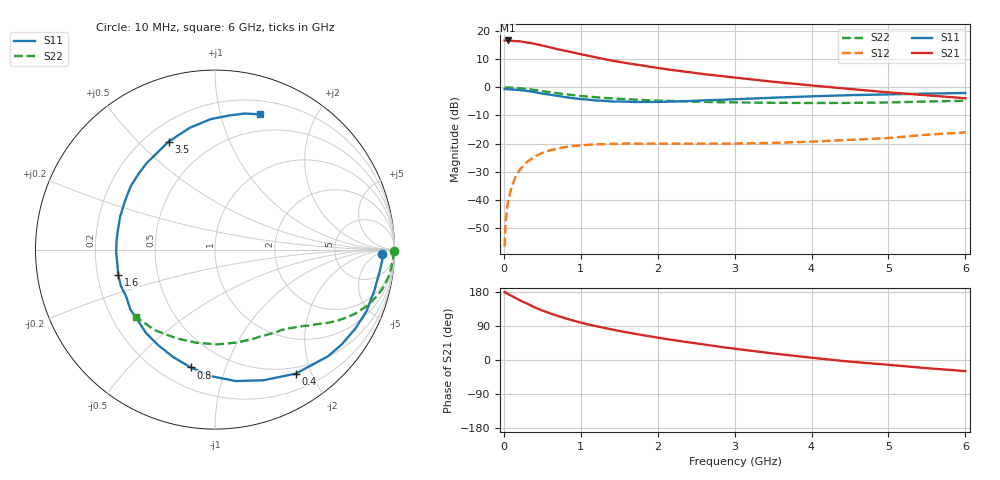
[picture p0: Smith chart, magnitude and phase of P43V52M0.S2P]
! SIEMENS Small Signal Semiconductors
! BFP182
! Si NPN RF Bipolar Junction Transistor in SOT143
! VCE = 3.5 V  IC = 2 mA
! Common Emitter S-Parameters:  March  1996
# GHz  S  MA  R  50
!  f  S11  S21  S12  S22
! GHz  MAG  ANG  MAG  ANG  MAG  ANG  MAG  ANG
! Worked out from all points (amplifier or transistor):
!   36 points, 10 MHz to 6 GHz, reference 50 ohm
!   highest |S21| = 16.7 dB at 50 MHz (marker M1)
!   |S21| within 3 dB of that: start of sweep to 680.8 MHz
!   unconditionally stable (mu >= 1): 2.2 GHz to 5.913 GHz
!   at 250 MHz: K = 0.12, MSG = 22.1 dB, |S12| = -27.9 dB
!   at 1.4 GHz: K = 0.68, MSG = 14.8 dB, |S12| = -20.1 dB
!   at 6 GHz: K = 0.99, MSG = 6.1 dB, |S12| = -16.0 dB
!   lowest NFmin = 1.10 dB at 450 MHz
!   S11 on the Smith chart (normalised r, x): 10 MHz: 25, -9; 400 MHz: 0.41, -1.77; 800 MHz: 0.32, -0.76; 1.6 GHz: 0.29, -0.12; 3.5 GHz: 0.29, +0.62; 6 GHz: 0.33, +1.33
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0.01  0.9308 -1.4  6.803 179.2  0.0015 85.8  0.9974 -0.5
0.02  0.9348 -3.1  6.801 178.4  0.0035 84.3  0.9896 -1.1
0.05  0.9259 -7.5  6.829 174.6  0.0088 88.7  0.9939 -2.8
0.1  0.9166 -14.7  6.738 169.3  0.0168 80.6  0.9872 -5.8
0.2  0.8968 -29.6  6.618 158.5  0.033 72.8  0.9678 -11.4
0.25  0.8817 -36.8  6.437 153.4  0.0401 68.8  0.953 -14.0
0.4  0.8248 -56.9  5.955 139.1  0.0588 58.0  0.8991 -20.7
0.5  0.7763 -69.7  5.545 130.5  0.0686 51.4  0.8582 -24.6
0.6  0.7414 -81.0  5.166 123.2  0.0759 46.0  0.8203 -27.7
0.7  0.7064 -91.5  4.759 116.4  0.0821 41.4  0.7876 -30.2
0.8  0.6705 -101.6  4.464 110.0  0.0869 36.8  0.7563 -32.5
0.9  0.6421 -111.4  4.178 104.1  0.0908 33.6  0.7288 -34.4
1.1  0.603 -129.6  3.654 93.6  0.0953 27.8  0.6834 -37.9
1.3  0.5776 -144.8  3.192 85.0  0.0978 23.3  0.6505 -40.8
1.6  0.5575 -165.3  2.696 73.0  0.1003 18.7  0.6166 -44.8
1.8  0.5507 -178.1  2.45 65.7  0.0999 17.1  0.5966 -47.5
2.2  0.5595 160.9  2.024 52.5  0.0999 14.1  0.573 -53.3
2.8  0.5999 135.1  1.604 35.1  0.0999 13.5  0.5442 -63.3
3.5  0.655 113.2  1.259 17.3  0.1029 14.5  0.5314 -77.3
4.5  0.7273 91.9  0.937 -4.4  0.1166 17.4  0.5293 -101.1
5.5  0.7756 77.8  0.723 -21.6  0.1442 17.9  0.5602 -126.7
6  0.7942 71.7  0.641 -29.3  0.1582 14.9  0.5782 -139.4
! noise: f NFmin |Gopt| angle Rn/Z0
0.45  1.1  0.42  29  0.36
0.9  1.2  0.4  58  0.3
1.8  1.85  0.32  126  0.22
